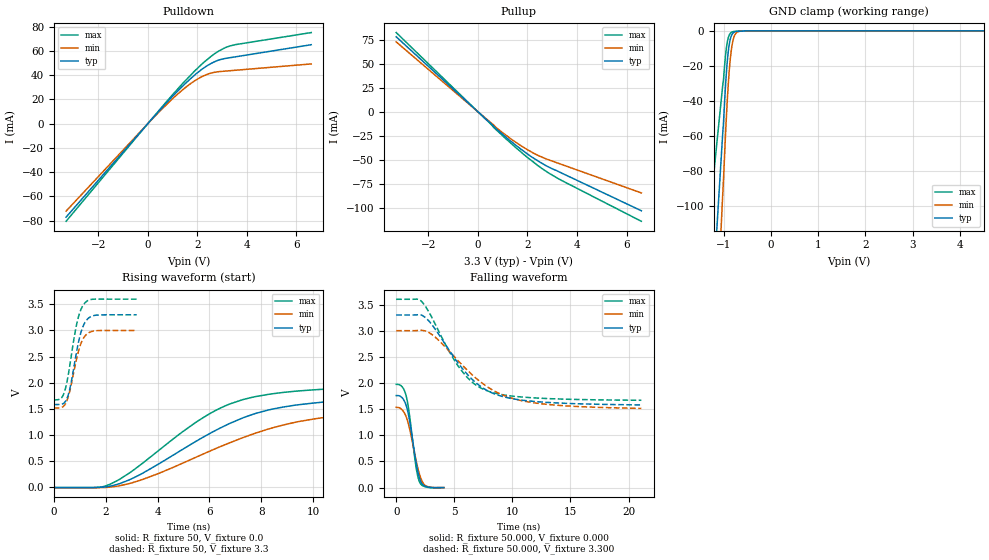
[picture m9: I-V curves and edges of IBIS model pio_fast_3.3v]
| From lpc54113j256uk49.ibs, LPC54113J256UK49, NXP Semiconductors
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[Model]   pio_fast_3.3v
Model_type I/O
Vinl=8.000E-01
Vinh=2.000E+00
Vref=0.000E+00
Rref=1.000E+06
Cref=2.000E-11
Vmeas=1.650E+00
C_comp   9.060E-12   8.700E-12   9.420E-12
[Voltage Range]   3.300E+00   3.000E+00   3.600E+00
[POWER Clamp Reference]   3.300E+00   3.000E+00   3.600E+00
[GND Clamp Reference]   0.000E+00   0.000E+00   0.000E+00
[Pullup Reference]   3.300E+00   3.000E+00   3.600E+00
[Pulldown Reference]   0.000E+00   0.000E+00   0.000E+00
[Temperature Range]   25   105   -40
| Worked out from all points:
|   slope of the pulldown table from 0 to 0.495 V, typ, clamps not added: 43.7 ohm
|   slope of the pullup table from 0 to 0.495 V, typ, clamps not added: 42.9 ohm
|   GND clamp passes 1 mA (typ) near -0.79 V on its own axis
|   rising waveform, R_fixture 50, V_fixture 0.0: 20-80 % time 4.01ns typ, 4.87ns min, 3.42ns max; typ from -0.007 V to 1.75 V
|   falling waveform, R_fixture 50.000, V_fixture 0.000: 20-80 % time 778ps typ, 900ps min, 693ps max; typ from 1.76 V to 0 V
|   rising waveform, R_fixture 50, V_fixture 3.3: 20-80 % time 406ps typ, 410ps min, 403ps max; typ from 1.58 V to 3.3 V
|   falling waveform, R_fixture 50.000, V_fixture 3.300: 20-80 % time 3.75ns typ, 4.6ns min, 3.19ns max; typ from 3.3 V to 1.58 V
[GND Clamp]
-3.3V     -1.057A    -1.379A    -638.8mA
-1.02V    -59.59mA   -94.78mA   -31.69mA
-1V       -51.98mA   -84.2mA    -27.5mA
-960mV    -32.15mA   -60.25mA   -14.52mA
-920mV    -17.1mA    -39.24mA   -6.27mA
-880mV    -7.792mA   -22.91mA   -2.41mA
-860mV    -5.008mA   -16.73mA   -1.493mA
-820mV    -1.972mA   -8.109mA   -648.8uA
-780mV    -812.3uA   -3.517mA   -349.3uA
-740mV    -402.4uA   -1.442mA   -243.8uA
-520mV    -16.02uA   -18.16uA   -14.02uA
6.6V      0A         0A         0A
[Power Clamp]
-3.3V     0A         0A         0A
0V        0A         0A         0A
3.3V      0A         0A         0A
6.6V      0A         0A         0A
[Pullup]
-3.3V     78.3mA     72.94mA    82.7mA
720mV     -17.43mA   -16.13mA   -18.38mA
1.36V     -31.35mA   -28.83mA   -33.53mA
1.82V     -40.62mA   -36.76mA   -43.91mA
2.5V      -52.53mA   -46.42mA   -57.65mA
3.22V     -62.03mA   -53.52mA   -69.47mA
6.6V      -103.4mA   -84.74mA   -114.4mA
[Pulldown]
-3.3V     -77.06mA   -72.09mA   -80.46mA
140mV     3.263mA    3.027mA    3.421mA
1.04V     23.4mA     21.38mA    24.81mA
1.46V     32mA       28.83mA    34.24mA
1.9V      40.22mA    35.44mA    43.55mA
2.22V     45.34mA    39.08mA    49.76mA
2.64V     50.5mA     42.1mA     56.82mA
3.12V     53.7mA     43.29mA    62.54mA
3.54V     55.09mA    44.01mA    65.14mA
6.6V      65.07mA    49.25mA    75.08mA
[Rising Waveform]
R_fixture = 50
V_fixture = 0.0
V_fixture_min = 0.0
V_fixture_max = 0.0
0s        -6.972mV   -11.77mV   -15.61mV
1.65ns    -6.031mV   -11.97mV   -9.955mV
2.2ns     18.82mV    -80.67uV   60.55mV
3.35ns    244.8mV    133.1mV    428.3mV
5.9ns     994.4mV    663.1mV    1.373V
6.8ns     1.222V     850.9mV    1.595V
7.8ns     1.413V     1.036V     1.735V
9.5ns     1.581V     1.26V      1.844V
11.85ns   1.674V     1.403V     1.905V
20.45ns   1.751V     1.522V     1.955V
[Falling Waveform]
R_fixture = 50.000
V_fixture = 0.000
V_fixture_min = 0.000
V_fixture_max = 0.000
|  time   V(typ)   V(min)   V(max)
0s        1.759V     1.535V     1.974V
550ps     1.708V     1.477V     1.916V
900ps     1.539V     1.329V     1.714V
1.15ns    1.28V      1.127V     1.376V
1.7ns     496mV      531.9mV    405.4mV
1.85ns    318.7mV    383.4mV    223.7mV
2ns       186.1mV    258.5mV    112.9mV
2.25ns    67.32mV    113mV      40.17mV
2.55ns    23.02mV    34.5mV     14.07mV
4.1ns     0V         0V         0V
[Rising Waveform]
R_fixture = 50
V_fixture = 3.3
V_fixture_min = 3.0
V_fixture_max = 3.6
0s        1.581V     1.514V     1.67V
300ps     1.587V     1.525V     1.711V
400ps     1.612V     1.559V     1.806V
500ps     1.688V     1.647V     1.996V
650ps     1.957V     1.914V     2.438V
900ps     2.65V      2.506V     3.163V
1.05ns    2.971V     2.756V     3.408V
1.2ns     3.154V     2.893V     3.529V
1.6ns     3.291V     2.993V     3.6V
3.2ns     3.3V       3V         3.6V
[Falling Waveform]
R_fixture = 50.000
V_fixture = 3.300
V_fixture_min = 3.000
V_fixture_max = 3.600
|  time   V(typ)   V(min)   V(max)
0s        3.3V       3V         3.6V
2.2ns     3.295V     3.007V     3.555V
3.2ns     3.078V     2.905V     3.196V
4.5ns     2.646V     2.624V     2.624V
5.4ns     2.36V      2.408V     2.303V
6.5ns     2.079V     2.164V     2.023V
7.65ns    1.878V     1.957V     1.866V
9.3ns     1.733V     1.758V     1.771V
11.7ns    1.651V     1.627V     1.718V
21.1ns    1.581V     1.514V     1.67V
[Ramp]
dV/dt_r   1.0546E+00/4.0018E-09   9.2039E-01/4.8626E-09   1.1824E+00/3.4156E-09
dV/dt_f   1.0315E+00/3.7458E-09   8.9139E-01/4.5835E-09   1.1580E+00/3.1818E-09
R_load = 50
